
FUNCTION FC 1 : VOID
TITLE =Send_Data

//Transfer FC for Siebert SX502 large size displays
//
//Inputs:
//SendDb        -> number of SendDB, this DB contains all parameters needed for
//                 data transmission to display
//                 Format of SendDB is:
//                 00     TxHsByte        // contains TxHsBit in bit 0
//                 01..63 Data area       // max 63 bytes for raw data
//                 64     NumOfSegments   // number of segments in data string
//                 66     SegmentCounter  // number of latest transmitted segment
//                 68     SourceDB        // number of Db for source string
//                 70     OutputAddr      // output start address
//                 72     InputAddr       // input address
//                 74     OutputLen       // configured length of output data
//Outputs:
//RETVAL:       -> = 0x0000 if transfer was ok.
//                 = 0x8000 if display was busy
//                 = 0x8001 if error in parameters (user error)
//                 = 0x8002 if DB not completely sent -> next segment must be sent
//                 = 0x8xxx if SFC15 or SFC20 failed (see S7 manual for details).
VERSION : 0.1


VAR_INPUT
  SendDb : WORD ;	//number of destination DB to be transmitted (also storage for TxHsByte)
END_VAR
VAR_OUTPUT
  RETVAL : INT ;	//0 if ok, error else (see description below)
END_VAR
VAR_TEMP
  T_AR1 : DWORD ;	//temp storage for AR1
  T_ANY_Source : ANY ;	//any pointer to source for SFC15
  T_ANY_Destination : ANY ;	//any pointer to destination for SFC20
  P_InputAddr : DWORD ;	//pointer to input data (i.e. RxHsByte) from display
  P_OutputAddr : DWORD ;	//pointer to output data from master
  T_SEND : WORD ;	//temp storage for number of SendDb
  T_DataLen : WORD ;	//number of bytes to be sent
  T_SRC : WORD ;	//temp storage for number of SrcDb
  T_TxStart : WORD ;	//temp storage for transmission start
  T_TxLen : WORD ;	//temp storage for transmission length
  T_TxSeg : WORD ;	//temp storage for segment to be sent
  P_Poi : DWORD ;	//temp general purpose pointer
END_VAR
BEGIN
NETWORK
TITLE =
//save AR1 contents to be restored upon exit of FC
      TAR1  #T_AR1; // save AR1 locally

NETWORK
TITLE =
//Open the SendDB and check display ready condition.
//

      L     W#16#0; // 0x0000 signals no error
      T     #RETVAL; // preset it here

      L     #SendDb; // get number of send data block
      L     W#16#0; // load compare value
      ==I   ; // number of SendDb equals 0 ?
      SPB   ERR; // no SendDb specified, signal error and quit

      L     #SendDb; // get number of send data block
      T     #T_SEND; // store locally
      AUF   DB [#T_SEND]; // open the send data block

      L     DBLG; // get length of SendDb
      L     W#16#4C; // get compare value
      ==I   ; // length of SendDb equals 76 ?
      SPBN  ERR; // no --> SendDb is no valid SendDb, signal error and quit

// ** get number of current segment
      L     DBW   64; // get number of segments stored in SendDB (SendDb.NumOfSegments)
      L     DBW   66; // get number of last segment sent from SendDb (SendDb.SegmentCounter)
      ==I   ; // equal ?
      SPB   EXIT; // nothing to send; jump out and signal ready for new data

      L     DBW   68; // get number of source data block (SendDb.SourceDB)
      T     #T_SRC; // store locally
      AUF   DB [#T_SRC]; // open the SourceDB; must contain data string beginning in byte 0 of DB
      L     DBB    1; // string length saved in 2nd byte of string i.e byte 1 of source DB
      T     #T_DataLen; // store data length locally
      AUF   DB [#T_SEND]; // open the send data block

// ** check display ready
// ** get TxHsBit and RxHsBit
      L     DBW   72; // get input address (RxHsByte from display) (SendDb.InputAddr)
      SLD   3; // convert to pointer format
      L     7; // point to bit 7
      +D    ;
      T     #P_InputAddr; // store locally

      CLR   ;
      U     E [#P_InputAddr]; // load RxHsBit
      U     DBX    0.0; // get previously sent TxHsBit (SendDb.TxHs)
      SPB   HS1; // both bits equal (set)? --> send allowed

      CLR   ;
      UN    E [#P_InputAddr]; // load RxHsBit
      UN    DBX    0.0; // get previously sent TxHsBit (SendDb.TxHs)
      SPB   HS0; // both bits equal (cleared)? --> send allowed

// ** handshake bits not equal i.e. display not ready for new data
      L     W#16#8000; // 0x8000 signals display busy
      T     #RETVAL; // set return value
      SPA   EXIT; // common exit

// ** toggle TxHsBit
HS1:  NOP   0; // hs bit set
      R     DBX    0.0; // clear TxHsBit and store in SendDb (SendDb.TxHs)
      SPA   SEND; // branch to send routine

HS0:  NOP   0; // hs bit cleared
      S     DBX    0.0; // set TxHsBit and store TxHsByte in SendDb (SendDb.TxHs)
      SPA   SEND; // branch to send routine

NETWORK
TITLE =
//Transmit data to display.
//Get total number of segments and number of current segment for transmission.
//Total number of segments and last segment are stored in SendDb.
//16 bit operation is ok for all calculations as maximum of data may not exceed
//2048 bytes (see SX502 manual).

SEND: NOP   0;
// ** clear data in send DB i.e. erase data from previous transmission
      L     DW#16#1; // load 1 to begin with byte 1 (erase SendDb Bytes 1 to 63)
      SLD   3; // convert to pointer format
      T     #P_Poi; // store tmp

Loop: L     B#16#0; // load 0 (erase value)
      T     DBB [#P_Poi]; // store in SendDb
      L     #P_Poi; // get value from pointer
      L     1; // load 1
      SLD   3; // pointer format
      +D    ; // add to pointer (i.e. increase pointer by one byte)
      T     #P_Poi; // store
      L     64; // load compare value
      SLD   3; // pointer format
      ==I   ; // compare
      SPBN  Loop; // loop if end not yet reached

// ** transfer data from source DB to send DB using SFC20
// ** assemble ANY-pointers for SFC20, then call SFC20

// ** calculate start and length of raw data
      L     DBW   66; // get number of last segment sent (SendDb.SegmentCounter) (equals 0 if no segment sent yet)
      L     DBW   74; // get length of consistent data (SendDb.OutputLen)
      +     L#-1; // dec consistent data length by 1 (HsByte) to get max length for raw data
      *I    ; // multiply to get start offset for data for next segment
      T     #T_TxStart; // store temp

      L     DBW   66; // get number of last segment sent from SendDb (SendDb.SegmentCounter)
      +     1; // inc number of sent segments by 1
      T     #T_TxSeg; // store tmp

      L     DBW   64; // load number of segments (SendDb.NumOfSegments)
      L     W#16#1; // load compare value 1
      ==I   ; // only 1 segment ?
      SPB   L320; // jump if true

      L     #T_TxSeg; // load number of current segment
      L     DBW   64; // load number of segments (SendDb.NumOfSegments)
      ==I   ; // current segment is last segment ?
      SPB   L330; // jump if true

      L     DBW   74; // not last segment, send as many bytes as possible (SendDb.OutputLen)
      +     L#-1; // dec consistent data length by 1 (HsByte) to get max length for raw data
      T     #T_TxLen; // store tmp
      SPA   L340;

L320: NOP   0; // only one segment to transmit
      L     #T_DataLen; // load data length
      T     #T_TxLen; // store tmp
      SPA   L340;

L330: NOP   0; // segment to transmit is last segment
      L     #T_DataLen; // load data length
      L     #T_TxStart; // get start offset for data
      -I    ; // substract offset from data length to get number of remaining bytes
      T     #T_TxLen; // store tmp

// ** copy data of current segment from SourceDB to data area of SendDB
// ** assemble ANY-pointer to source DB for SFC20
L340: NOP   0;
      LAR1  P##T_ANY_Source;

      L     W#16#1002; // syntax ID is (10hex) for ANY pointer in S7; type is byte (02hex)
      T     LW [AR1,P#0.0]; // store in ANY pointer

      L     #T_TxLen; // get length in bytes
      T     LW [AR1,P#2.0]; // store in ANY pointer

      L     DBW   68; // load number of source DB (SendDb.SourceDB)
      T     LW [AR1,P#4.0]; // store in ANY pointer

      AUF   DB [#T_SRC]; // open source DB
      L     P#DBX 2.0; // load pointer to start of data (raw data in string starts in 3rd byte i.e. Addr 2.0 of SourceDB)
      L     #T_TxStart; // load start position offset in source DB
      SLD   3; // convert to pointer format
      +D    ; // add to pointer to source DB
      T     LD [AR1,P#6.0]; // store in ANY pointer

// ** assemble ANY-pointer to SendDb for SFC 20
      LAR1  P##T_ANY_Destination;

      L     W#16#1002; // syntax ID is (10hex) for ANY pointer in S7; type is byte (02hex)
      T     LW [AR1,P#0.0]; // store in ANY pointer

      L     #T_TxLen; // get length in bytes
      T     LW [AR1,P#2.0]; // store in ANY pointer

      L     #SendDb; // store number of SendDb (input to function)
      T     LW [AR1,P#4.0]; // store in ANY pointer

      AUF   DB [#T_SEND]; // open SendDb
      L     P#DBX 0.0; // load pointer to start of SendDb
      L     W#16#1; // load start position in SendDb
      SLD   3; // convert to pointer format
      +D    ; // add to pointer to SendDb
      T     LD [AR1,P#6.0]; // store in ANY pointer

// ** copy raw data to SendDb; use SFC 20
      CALL SFC   20 (
           SRCBLK                   := #T_ANY_Source,
           RET_VAL                  := #RETVAL,
           DSTBLK                   := #T_ANY_Destination);

      L     #RETVAL; // get return value from function
      L     W#16#0; // load compare value 0
      ==I   ; // equal ?
      SPBN  EXIT; // No! --> error occured; jump out

// ** if data successfully copied to SendDb, transfer SendDb to output data area
// ** take care of consistency over whole length of data
// ** 2 or 4 bytes can be transferred directly, use SFC 15 else

// ** get output data address
      L     DBW   70; // get output address start (SendDb.OutputAddr)
      SLD   3; // convert to pointer format
      T     #P_OutputAddr; // store locally

      L     DBW   74; // get length of consistent data (SendDb.OutputLen)
      L     W#16#2; // get  compare value
      ==I   ; // length of consistent data equals 2 ?
      SPB   Tx2; // transmit 2 bytes

      L     DBW   74; // get length of consistent data (SendDb.OutputLen)
      L     W#16#4; // get  compare value
      ==I   ; // length of consistent data equals 4 ?
      SPB   Tx4; // transmit 4 bytes

// ** consistent transmission of 3 or more than 4 bytes needs SFC 15
// ** assemble ANY-pointer to SendDb for SFC15

      LAR1  P##T_ANY_Destination;

      L     W#16#1002; // syntax ID is (10hex) for ANY pointer in S7; type is byte (02hex)
      T     LW [AR1,P#0.0]; // store in ANY pointer

      L     DBW   74; // get length in bytes (SendDb.OutputLen)
      T     LW [AR1,P#2.0]; // store in ANY pointer

      L     #SendDb; // store number of SendDb (input to function)
      T     LW [AR1,P#4.0]; // store in ANY pointer

      L     P#DBX 0.0; // load pointer to start of SendDb
      T     LD [AR1,P#6.0]; // store in ANY pointer

      CALL SFC   15 (// call SIEMENS SFC for consistent byte transfer
           LADDR                    := DBW   70,// output bytes assigned to converter (SendDb.OutputAddr)
           RECORD                   := #T_ANY_Destination,// any pointer for source data (see above)
           RET_VAL                  := #RETVAL);// return value form SFC (0 if ok, see manual for error messages else)

      L     #RETVAL; // get return value from function
      L     W#16#0; // load compare value 0
      ==I   ; // equal ?
      SPBN  EXIT; // No! --> error occured; jump out
      SPA   SAVE; // transmission finished

Tx2:  NOP   0;
      L     DBW    0; // read word (2 bytes) from SendDb
      T     AW [#P_OutputAddr]; // write to converter (S7300 assures consitency)
      SPA   SAVE; // transmission finished

Tx4:  NOP   0;
      L     DBD    0; // read double word (4 bytes) from SendDb
      T     AD [#P_OutputAddr]; // write to converter (S7300 assures consitency)
      SPA   SAVE; // transmission finished

// ** transmission completed
SAVE: NOP   0; // store segment number after successful transmission
      L     #T_TxSeg; // get number of segment just sent
      T     DBW   66; // store in send DB (SendDb.SegmentCounter)
      L     DBW   64; // load total number of segments (SendDb.NumOfSegments)
      ==I   ; // sent segment equals last segment ?
      SPB   EXIT; // ok done, leave with result = 0x0000

      L     W#16#8002; // load error condition 0x8002, sending source DB not yet completed
      T     #RETVAL; // store in return value
      SPA   EXIT; // ok done, leave with result = 0x8002

ERR:  NOP   0; // set error 0x8001 (error in parameters)
      L     W#16#8001;
      T     #RETVAL;
      SPA   EXIT; // leave with result = 0x8001

NETWORK
TITLE =
//Restore original value of AR1
EXIT: NOP   0; // common exit point

      LAR1  #T_AR1; // restore value of AR1
      BE    ;


END_FUNCTION

